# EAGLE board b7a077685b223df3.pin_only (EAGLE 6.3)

Size 22.86 x 20.97 mm. Coordinates in mm from the lower left corner, seen from the top.
Outline: 0,2.54 0,18.43 arc-90 2.54,20.97 20.32,20.97 arc-90 22.86,18.43 22.86,2.54 arc-90 20.32,0 2.54,0 arc-90 0,2.54
Copper layers (1*16): Top 0.035mm / dielectric 1.5mm / Bottom 0.035mm
Design rules "default": minimum track width 8mil, minimum drill 0.4mm, track to track 8mil, track to pad 8mil, pad to pad 8mil, via to via 8mil, smd to smd 8mil, copper to edge 20mil, drill to drill 8mil, minimum pad ring 8mil, minimum via ring 10mil, stop-mask expansion 3mil, vias tented up to drill 20mil, thermal gap 8mil

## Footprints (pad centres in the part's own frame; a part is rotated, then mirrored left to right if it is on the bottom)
0805 = smd 1.3 x 1.5: 1 -0.95,0; 2 0.95,0
FIDUCIAL_1MM = smd 1 x 1: 1 0,0
TERMBLOCK_1X2-3.5MM = drill 1 pad 2.184: 1 1.8,0; 2 -1.7,0
1X05_ROUND_70 = drill 1 pad 1.778 square: 1 -5.08,0 | drill 1 pad 1.778: 2 -2.54,0; 3 0,0; 4 2.54,0; 5 5.08,0
0805-THM = drill 0.813 pad 1.676 octagon: 1 -5.08,0; 2 5.08,0
2512 = smd 1.8 x 3.2: 1 -2.8,0; 2 2.8,0
SOT23-5 = smd 0.55 x 1.2: 1 -0.95,-1.3; 2 0,-1.3; 3 0.95,-1.3; 4 0.95,1.3; 5 -0.95,1.3
MOUNTINGHOLE_2.5_PLATED = drill 2.5 pad 3.2: P$1 0,0

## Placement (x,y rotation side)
C1  0.1µF  [0805]  5.33,12.12 180 top
FID1  FIDUCIAL""  [FIDUCIAL_1MM]  17.93,15.96 0 top
FID2  FIDUCIAL""  [FIDUCIAL_1MM]  2.54,5.84 0 top
J1  [TERMBLOCK_1X2-3.5MM]  11.4,17.38 180 top
JP1  [1X05_ROUND_70]  11.43,2.54 0 top
R1  10K  [0805-THM]  21.34,10.41 90 top
RSHUNT  0.1/1% (PT2512FK-070R1L)  [2512]  11.43,11.51 0 top
U1  INA169  [SOT23-5]  11.43,7.37 90 top
U$7  MOUNTINGHOLE2.5  [MOUNTINGHOLE_2.5_PLATED]  20.32,2.54 0 top
U$8  MOUNTINGHOLE2.5  [MOUNTINGHOLE_2.5_PLATED]  2.54,2.54 0 top
U$9  MOUNTINGHOLE2.5  [MOUNTINGHOLE_2.5_PLATED]  2.54,18.43 0 top
U$10  MOUNTINGHOLE2.5  [MOUNTINGHOLE_2.5_PLATED]  20.32,18.43 0 top
U$11  [ADAFRUIT_3.5MM]  3.33,6.68 0 top

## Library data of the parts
C1 J1 JP1 R1 RSHUNT U1 U$7-U$11 = microbuilder
FID1 FID2 = microbuilder; BOM: EXCLUDE

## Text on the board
tPlace: Vin- | Vin+ | Rshunt | INA169 | Load Resistor | VCC | VIN- | OUT | GND | VIN+
bPlace: INA169 DC | Current Sensor | VCC/VIN: 2.7-60V | Max Current: 5A | Vout=RL/10K*I(Amps)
